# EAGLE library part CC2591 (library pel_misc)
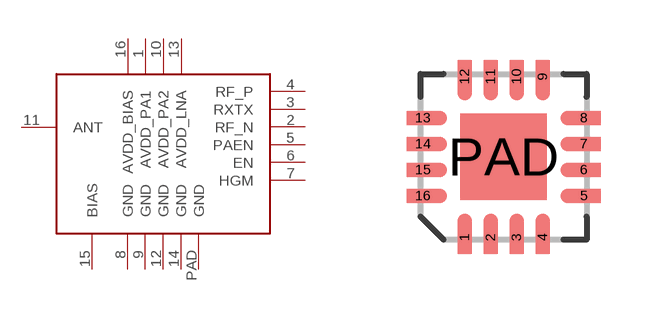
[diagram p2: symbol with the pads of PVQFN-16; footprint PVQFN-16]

Designator prefix IC

## CC2591  [PVQFN-16]
1  AVDD_PA1
2  RF_N
3  RXTX
4  RF_P
5  PAEN
6  EN
7  HGM
8  GND
9  GND
10  AVDD_PA2
11  ANT
12  GND
13  AVDD_LNA
14  GND
15  BIAS
16  AVDD_BIAS
PAD  GND

## Footprint PVQFN-16 (pad centres in mm)
smd 0.35 x 0.825: 1 -0.975,-2.013; 2 -0.325,-2.013; 3 0.325,-2.013; 4 0.975,-2.013; 9 0.975,2.013; 10 0.325,2.013; 11 -0.325,2.013; 12 -0.975,2.013
smd 0.825 x 0.35: 5 2.013,-0.975; 6 2.013,-0.325; 7 2.013,0.325; 8 2.013,0.975; 13 -2.013,0.975; 14 -2.013,0.325; 15 -2.013,-0.325; 16 -2.013,-0.975
smd 2.16 x 2.16: PAD 0,0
